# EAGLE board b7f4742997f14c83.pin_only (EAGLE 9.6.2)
REV: C

Size 43.18 x 27.94 mm. Coordinates in mm from the lower left corner, seen from the top.
Outline: 0,2.54 0,25.4 arc-90 2.54,27.94 40.64,27.94 arc-90 43.18,25.4 43.18,2.54 arc-90 40.64,0 2.54,0 arc-90 0,2.54
Copper layers (1*16): Top 0.035mm / dielectric 1.5mm / Bottom 0.035mm
Design rules "adafruit *": minimum track width 7mil, minimum drill 15.5mil, track to track 7mil, track to pad 8mil, pad to pad 8mil, via to via 8mil, smd to smd 8mil, copper to edge 10mil, drill to drill 8mil, minimum pad ring 10mil, minimum via ring 8mil, stop-mask expansion 2mil, vias tented up to drill 20mil, thermal gap 10mil
tRestrict: area 27.2,12.6 to 35.4,14.9

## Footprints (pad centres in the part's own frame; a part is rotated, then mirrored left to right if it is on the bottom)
0805-NO = smd 1.24 x 1.5: 1 -0.95,0; 2 0.95,0
0603-NO = smd 1.075 x 1: 1 -0.85,0; 2 0.85,0
JST_SH4 = smd 0.6 x 1.55: 1 -1.5,2.006; 2 -0.5,2.006; 3 0.5,2.006; 4 1.5,2.006 | smd 1.2 x 1.8: MT1 -2.8,-1.894; MT2 2.8,-1.894
FIDUCIAL_1MM = smd 1 x 1: 1 0,0
1X13_ROUND_70 = drill 1 pad 1.676: 1 -15.24,0; 2 -12.7,0; 3 -10.16,0; 4 -7.62,0; 5 -5.08,0; 6 -2.54,0; 7 0,0; 8 2.54,0; 9 5.08,0; 10 7.62,0; 11 10.16,0; 12 12.7,0; 13 15.24,0
1X07_ROUND_76 = drill 1 pad 1.93: 1 -7.62,0; 2 -5.08,0; 3 -2.54,0; 4 0,0; 5 2.54,0; 6 5.08,0; 7 7.62,0
0603-THM = drill 0.813 pad 1.676 octagon: 1 -5.08,0; 2 5.08,0 | smd 1.075 x 1: 11 -0.85,0; 22 0.85,0
SOLDERJUMPER_ARROW_NOPASTE = smd 0.762 x 1.524: 1 -1.016,0; 2 1.016,0
QFN28_4MM_0.4MM = smd 0.6 x 0.18: 1 -2,1.2; 2 -2,0.8; 3 -2,0.4; 4 -2,0; 5 -2,-0.4; 6 -2,-0.8; 7 -2,-1.2; 15 2,-1.2; 16 2,-0.8; 17 2,-0.4; 18 2,0; 19 2,0.4; 20 2,0.8; 21 2,1.2 | smd 0.18 x 0.6: 8 -1.2,-2; 9 -0.8,-2; 10 -0.4,-2; 11 0,-2; 12 0.4,-2; 13 0.8,-2; 14 1.2,-2; 22 1.2,2; 23 0.8,2; 24 0.4,2; 25 0,2; 26 -0.4,2; 27 -0.8,2; 28 -1.2,2 | smd 2.3 x 2.3: THERMAL 0,0
MOUNTINGHOLE_2.5_PLATED = drill 2.5 pad 3.2: P$1 0,0

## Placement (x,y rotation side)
C1  10uF  [0805-NO]  33.15,8.64 270 top
C2  0.1uF  [0603-NO]  17.91,18.54 180 top
C3  0.22uF  [0603-NO]  35.69,8.13 270 top
C4  10uF  [0805-NO]  6.6,18.8 270 top
C5  0.1uF  [0603-NO]  26.16,9.14 0 top
CONN1  STEMMA_I2C_QT  [JST_SH4]  40.01,17.78 90 top
CONN2  STEMMA_I2C_QT  [JST_SH4]  40.01,10.16 90 top
FID1  FIDUCIAL_1MM  [FIDUCIAL_1MM]  39.24,22.23 180 top
FID2  FIDUCIAL_1MM  [FIDUCIAL_1MM]  14.99,13.34 180 top
JP2  [1X13_ROUND_70]  21.59,26.67 0 top
JP4  [1X13_ROUND_70]  21.59,1.27 0 top
JP5  [1X07_ROUND_76]  2.54,13.97 270 top
PLABEL0  [PLABEL0]  6.6,2.79 0 top
PLABEL1  [PLABEL1]  9.14,2.79 0 top
PLABEL2  [PLABEL2]  11.68,2.79 0 top
PLABEL3  [PLABEL3]  14.22,2.79 0 top
PLABEL4  [PLABEL4]  16.76,2.79 0 top
PLABEL5  [PLABEL5]  19.3,2.79 0 top
PLABEL6  [PLABEL6]  21.84,2.79 0 top
PLABEL7  [PLABEL7]  24.38,2.79 0 top
PLABEL8  [PLABEL8]  26.92,2.79 0 top
PLABEL9  [PLABEL9]  16.51,25.15 0 top
PLABEL10  [PLABEL10]  19.05,25.15 0 top
PLABEL11  [PLABEL11]  21.59,25.15 0 top
PLABEL12  [PLABEL12]  24.13,25.15 0 top
PLABEL13  [PLABEL13]  26.67,25.15 0 top
PLABEL14  [PLABEL14]  29.21,25.15 0 top
PLABEL15  [PLABEL15]  31.75,25.15 0 top
PLABEL16  [PLABEL16]  34.29,25.15 0 top
PLABEL17  [PLABEL17]  36.83,25.15 0 top
PLABEL18  [PLABEL18]  31.75,4.06 90 top
PLABEL19  [PLABEL19]  29.21,4.83 90 top
PLABEL20  [PLABEL20]  36.83,4.7 90 top
PLABEL21  [PLABEL21]  34.29,4.32 90 top
PLABEL22  [PLABEL22]  30.61,19.43 0 top
PLABEL23  [PLABEL23]  5.71,25.65 270 top
PLABEL24  [PLABEL24]  8.38,25.65 270 top
PLABEL25  [PLABEL25]  10.92,25.65 270 top
PLABEL26  [PLABEL26]  13.46,25.65 270 top
PLABEL27  [PLABEL27]  4.83,20.07 90 top
PLABEL28  [PLABEL28]  1.27,17.27 90 top
PLABEL29  [PLABEL29]  4.83,15.11 90 top
PLABEL30  [PLABEL30]  1.27,12.7 90 top
PLABEL31  [PLABEL31]  4.32,11.68 90 top
PLABEL32  [PLABEL32]  0.76,9.02 90 top
PLABEL33  [PLABEL33]  4.57,6.35 90 top
PLABEL34  [PLABEL34]  19.68,7.37 0 top
PLABEL35  [PLABEL35]  10.67,6.73 90 top
PLABEL36  [PLABEL36]  8.13,6.73 90 top
PLABEL37  [PLABEL37]  13.34,6.73 90 top
PLABEL38  [PLABEL38]  30.1,11.43 0 top
PLABEL39  [PLABEL39]  7.62,14.22 0 top
R1  20K  [0603-THM]  31.5,13.72 180 top
R2  20K  [0603-NO]  29.72,9.65 270 top
R3  20K  [0603-NO]  10.03,18.8 90 top
R4  20K  [0603-NO]  8.51,18.8 90 top
R5  20K  [0603-NO]  31.24,9.65 90 top
R6  20K  [0603-NO]  12.95,16.76 0 top
SJ1  [SOLDERJUMPER_ARROW_NOPASTE]  12.83,12.19 90 top
SJ2  [SOLDERJUMPER_ARROW_NOPASTE]  7.62,12.19 90 top
SJ3  [SOLDERJUMPER_ARROW_NOPASTE]  10.16,12.19 90 top
U1  IS31FL3731-SALS2  [QFN28_4MM_0.4MM]  21.59,13.97 135 top
U$3  MOUNTINGHOLE2.5  [MOUNTINGHOLE_2.5_PLATED]  2.54,2.54 180 top
U$4  MOUNTINGHOLE2.5  [MOUNTINGHOLE_2.5_PLATED]  40.64,2.54 180 top
U$5  MOUNTINGHOLE2.5  [MOUNTINGHOLE_2.5_PLATED]  2.54,25.4 180 top
U$6  MOUNTINGHOLE2.5  [MOUNTINGHOLE_2.5_PLATED]  40.64,25.4 180 top
U$10  [ADAFRUIT_5MM]  16.76,19.18 0 top
U$11  [PCBFEAT-REV-040]  27.18,11.05 0 top

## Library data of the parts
C1-C5 JP2 JP4 JP5 R1-R6 U$10 = microbuilder
CONN1 CONN2 = adafruit_electromech; LCSC: C2845363
FID1 FID2 SJ1-SJ3 = microbuilder; BOM: EXCLUDE
PLABEL0 PLABEL1-PLABEL39 = pinguin
U1 = microbuilder; ROT: 270
U$3-U$6 = adafruit_electromech; BOM: EXCLUDE
U$11 = microbuilder; REV: C

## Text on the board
Pinguin_tBackup: VCC | GND | SCL | SDA | B1 | B2 | B3 | B4 | B5 | B6 | B7 | B8 | B9 | VCC | GND | IS31FL3731 / PWM LED / I2C Driver | SCL | SDA | I2C addr | AUD | Rext | INTB | 0x75 | 0x76 | 0x77 | 9x16 LED / Matrix Driver / Vcc: 2.7-5.5V | !SD | !SHUTD | AUDIO | INTB | ADDR | A1 | A2 | A3 | A4 | A5 | A6 | A7 | A8 | A9

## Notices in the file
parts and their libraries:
microbuilder: This work is placed in the public domain, and may be freely used for commercial and non-commercial work with the following conditions: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
